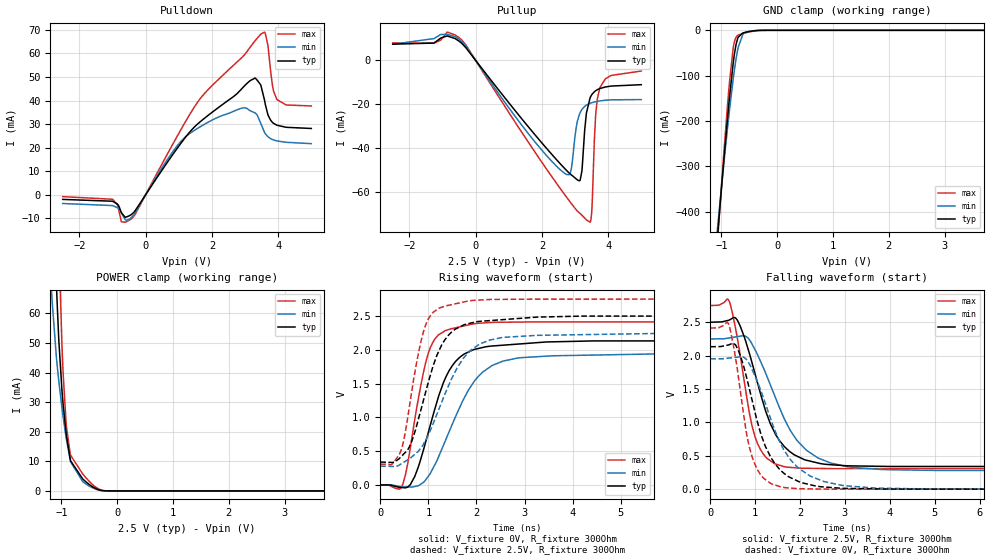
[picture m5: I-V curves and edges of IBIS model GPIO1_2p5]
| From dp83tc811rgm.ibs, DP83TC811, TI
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|   GPIO1_2p5 Model
[Model]   GPIO1_2p5
Model_type   I/O
Polarity   Non-Inverting
Enable   Active-Low
Vinl = 0.7
Vinh = 1.7
Vmeas = 1.25
Vref = 0
Cref = 2pF
Rref = 100000
|   typ   min   max
C_comp   7.4075pF   5.3413pF   9.7648pF
| Where Nom  PVT is Nominal Process, 2.5V, 27C
|   Fast PVT is Strong Process,  2.75V, -40C
|   Slow PVT is Weak Process,   2.25V, 125C
[Voltage Range]   2.5   2.25   2.75
|Junction Temperature
[Temperature Range]   27   125   -40
[Pullup Reference]   2.5   2.25   2.75
[Pulldown Reference]   0   0   0
[Power Clamp Reference]   2.5   2.25   2.75
[GND Clamp Reference]   0   0   0
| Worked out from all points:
|   slope of the pulldown table from 0 to 0.375 V, typ, clamps not added: 47.1 ohm
|   slope of the pullup table from 0 to 0.375 V, typ, clamps not added: 51.4 ohm
|   GND clamp passes 1 mA (typ) near -0.41 V on its own axis
|   POWER clamp passes 1 mA (typ) near -0.41 V on its own axis
|   falling waveform, V_fixture 2.5V, R_fixture 300Ohm: 20-80 % time 645ps typ, 855ps min, 390ps max; typ from 2.5 V to 0.339 V
|   rising waveform, V_fixture 0V, R_fixture 300Ohm: 20-80 % time 586ps typ, 790ps min, 382ps max; typ from 0 V to 2.13 V
|   rising waveform, V_fixture 2.5V, R_fixture 300Ohm: 20-80 % time 562ps typ, 759ps min, 371ps max; typ from 0.339 V to 2.5 V
|   falling waveform, V_fixture 0V, R_fixture 300Ohm: 20-80 % time 600ps typ, 774ps min, 363ps max; typ from 2.13 V to 0 V
[Pulldown]
|   Voltage   I(typ)   I(min)   I(max)
-2.5V     -1.936mA   -3.679mA   -766uA
-1.008V   -2.705mA   -4.545mA   -1.872mA
-730mV    -7.624mA   -7.561mA   -11.44mA
-430mV    -8.372mA   -9.666mA   -10.17mA
852.5mV   17.75mA    18.92mA    22.3mA
1.482V    28.92mA    27.44mA    37.52mA
3.305V    49.58mA    34.76mA    65.42mA
3.59V     40.06mA    26.43mA    69.07mA
3.695V    33.83mA    24.6mA     62.93mA
3.83V     30.71mA    23.45mA    46.18mA
3.958V    29.58mA    22.89mA    40.56mA
5V        28.16mA    21.72mA    37.72mA
[GND Clamp]
|   Voltage   I(typ)   I(min)   I(max)
-2.5V     -2.764A    -2.404A    -3.114A
-1.15V    -576.9mA   -538.8mA   -605.4mA
-1.052V   -427.7mA   -413mA     -433.2mA
-1.045V   -416.4mA   -403.5mA   -420.1mA
-940mV    -262.2mA   -273.4mA   -242.5mA
-857.5mV  -150.4mA   -177.8mA   -116.5mA
-782.5mV  -65.55mA   -100.6mA   -34.03mA
-737.5mV  -30.88mA   -62.27mA   -14.86mA
-700mV    -15.26mA   -37.35mA   -10.41mA
-602.5mV  -5.301mA   -7.441mA   -6.585mA
-362.5mV  -448.9uA   -368.7uA   -675.1uA
5V        0A         0A         0A
[Pullup]
|   Voltage   I(typ)   I(min)   I(max)
-2.5V     7.343mA    7.313mA    7.913mA
-445mV    8.07mA     8.896mA    9.631mA
2.728V    -49.78mA   -51.71mA   -61.82mA
2.877V    -51.91mA   -50.09mA   -64.85mA
3.125V    -54.73mA   -24.84mA   -69.22mA
3.208V    -50.3mA    -22.33mA   -70.37mA
3.342V    -24.03mA   -20.35mA   -72.47mA
3.455V    -17.02mA   -19.51mA   -73.54mA
3.515V    -15.42mA   -19.21mA   -65.73mA
3.62V     -13.84mA   -18.81mA   -25.52mA
3.748V    -12.83mA   -18.46mA   -12.55mA
5V        -11.07mA   -17.84mA   -4.855mA
[POWER Clamp]
|   Voltage   I(typ)   I(min)   I(max)
-2.5V     1.336A     1.089A     1.531A
-1.173V   120.8mA    65.99mA    187.7mA
-1.083V   66.33mA    43.57mA    110.8mA
-1.045V   50.26mA    36.74mA    82.68mA
-992.5mV  34.39mA    28.38mA    50.31mA
-970mV    29.3mA     25.1mA     39.83mA
-917.5mV  19.8mA     18.15mA    23.26mA
-842.5mV  10.72mA    10.39mA    12.48mA
-617.5mV  4.019mA    3.114mA    5.71mA
-445mV    1.425mA    1.073mA    2.195mA
-145mV    6.63uA     8.323uA    11.52uA
5V        0A         0A         0A
[Ramp]
R_load = 300
|   typ   min   max
dV/dt_r   1.28022/5.83999e-10   1.17212/7.88238e-10   1.44784/3.80118e-10
dV/dt_f   1.29669/6.41499e-10   1.18281/8.43786e-10   1.46551/3.87726e-10
[Falling Waveform]
V_fixture = 2.5V
V_fixture_min = 2.25V
V_fixture_max = 2.75V
R_fixture = 300Ohm
C_fixture = 0F
|   Time   V(typ)   V(min)   V(max)
0s        2.5V       2.25V      2.75V
399.5ps   2.528V     2.263V     2.842V
594.7ps   2.54V      2.284V     2.294V
871.7ps   2.034V     2.237V     1.14V
1.007ns   1.706V     2.077V     766.6mV
1.339ns   978.7mV    1.561V     425.7mV
1.635ns   651mV      1.076V     339.1mV
2.385ns   394.2mV    473.3mV    310.7mV
3.843ns   341.7mV    293.2mV    307.6mV
20ns      338.8mV    278.6mV    307.4mV
[Rising Waveform]
V_fixture = 0V
V_fixture_min = 0V
V_fixture_max = 0V
R_fixture = 300Ohm
C_fixture = 0F
|   Time   V(typ)   V(min)   V(max)
0s        60.08uV    69.93uV    138.6uV
469.8ps   -39.54mV   -28.88mV   12.49mV
716.1ps   124.6mV    -23.44mV   962.9mV
946.2ps   643.3mV    77.82mV    1.817V
1.099ns   1.038V     251.7mV    2.119V
1.433ns   1.692V     789.6mV    2.301V
1.918ns   1.995V     1.495V     2.381V
2.554ns   2.068V     1.833V     2.407V
3.576ns   2.117V     1.91V      2.412V
20ns      2.134V     1.954V     2.413V
[Rising Waveform]
V_fixture = 2.5V
V_fixture_min = 2.25V
V_fixture_max = 2.75V
R_fixture = 300Ohm
C_fixture = 0F
|   Time   V(typ)   V(min)   V(max)
0s        338.8mV    278.6mV    307.4mV
236.9ps   332.9mV    273.9mV    303mV
440.2ps   423mV      314.6mV    528.9mV
606.9ps   566.3mV    388.3mV    1.166V
805.2ps   1.006V     511.1mV    1.991V
1.001ns   1.526V     743mV      2.458V
1.331ns   2.135V     1.322V     2.642V
1.822ns   2.385V     1.948V     2.72V
3.254ns   2.483V     2.213V     2.749V
20ns      2.5V       2.25V      2.75V
[Falling Waveform]
|Gnd
V_fixture = 0V
V_fixture_min = 0V
V_fixture_max = 0V
R_fixture = 300Ohm
C_fixture = 0F
|   Time   V(typ)   V(min)   V(max)
0s        2.133V     1.952V     2.413V
404.5ps   2.16V      1.963V     2.48V
564.6ps   2.159V     1.974V     1.959V
800.3ps   1.696V     1.947V     867.7mV
944.4ps   1.298V     1.772V     461.8mV
1.227ns   642.5mV    1.284V     144mV
1.593ns   267.7mV    648.2mV    30.8mV
2.236ns   65.21mV    193mV      4.211mV
3.707ns   4.45mV     15.63mV    602.7uV
20ns      58.03uV    69.3uV     135.6uV
